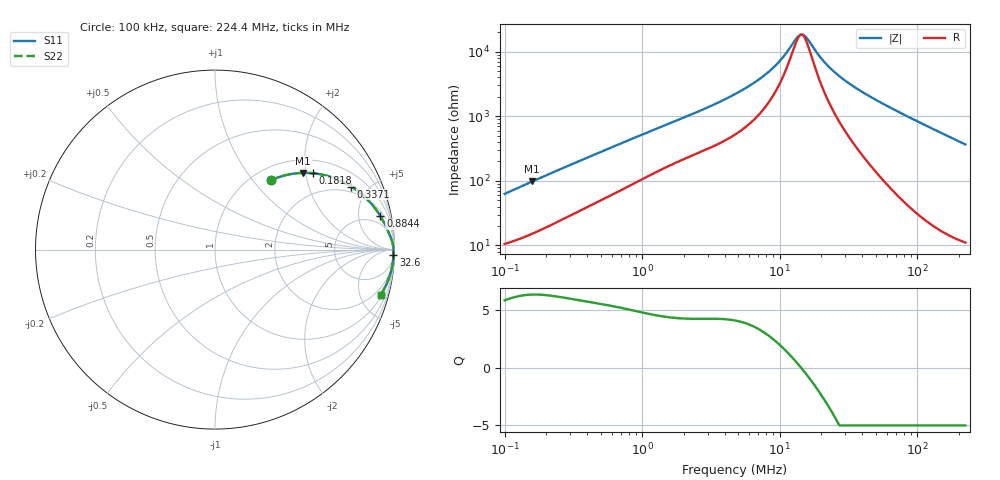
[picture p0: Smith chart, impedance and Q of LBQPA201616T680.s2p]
! LBQPA201616T680  S-PARAMETER MODEL  ( General Type )
! Model Generated by TAIYO YUDEN Corporation (http://www.ty-top.com)
! Version 1.0
! TAIYO YUDEN Control No. 191025NI43SB-FBB
! Copyright(c) 2019 TAIYO YUDEN CO.,LTD. All Rights Reserved.
! Product Description (link to TY-COMPAS)
! https://ds.yuden.co.jp/TYCOMPAS/or/detail?pn=LBQPA201616T680K&u=M
! Products Name : Inductors
! Characteristics :
!  Inductance : 68 uH , SRF(min) : 10 MHz , DC Resistance(max) : 9.1 Ohm
!  Rated Current : Saturation :130 mA , Temp Rise : 105 mA (20 degC)
!  Case Size : 2.0 x 1.6 / 0.079 x 0.063 [mm/inch] , Thickness : 1.6 / 0.063 [mm/inch]
!  (Conditions: Temperature = 25 degC , DC Bias Current/Voltage = 0A / 0V)
! External Node Assignments :
!  1  o---GGG---o  2
! GND o---------o GND
! Frequency Range : 0.1MHz  -  224.402193MHz  [ 402 STEP ]
# MHz S RI R 50
! Freq[MHz].  S11 Real  S11 Imag  S21 Real  S21 Imag  S12 Real  S12 Imag  S22 Real  S22 Imag
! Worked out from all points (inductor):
!   401 points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, 100 kHz to 224.4 MHz, reference 50 ohm
!   read as one part in series: L = 97.8 uH near 103.9 kHz
!   highest Q = 6.37 at 158.9 kHz (marker M1), where L = 96.9 uH
!   self-resonance near 14.22 MHz
!   S11 on the Smith chart (normalised r, x): 100 kHz: 1.21, +1.24; 181.8 kHz: 1.35, +2.20; 337.1 kHz: 1.66, +3.87; 884.4 kHz: 2.85, +9.15; 32.6 MHz: 10, -62; 224.4 MHz: 1.22, -7.31
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0.1  0.3117 0.3857  0.6883 -0.3857  0.6883 -0.3857  0.3117 0.3857
0.158877  0.4909 0.4275  0.5091 -0.4275  0.5091 -0.4275  0.4909 0.4275
0.181846  0.5459 0.4255  0.4541 -0.4255  0.4541 -0.4255  0.5459 0.4255
0.337122  0.7592 0.3512  0.2408 -0.3512  0.2408 -0.3512  0.7592 0.3512
0.364164  0.7795 0.3377  0.2205 -0.3377  0.2205 -0.3377  0.7795 0.3377
0.556677  0.8664 0.2607  0.1336 -0.2607  0.1336 -0.2607  0.8664 0.2607
0.884433  0.922 0.1857  0.078 -0.1857  0.078 -0.1857  0.922 0.1857
1.326154  0.9494 0.1349  0.0506 -0.1349  0.0506 -0.1349  0.9494 0.1349
2.868777  0.9778 0.0711  0.0222 -0.0711  0.0222 -0.0711  0.9778 0.0711
4.737111  0.9875 0.0431  0.0125 -0.0431  0.0125 -0.0431  0.9875 0.0431
6.575552  0.9912 0.0283  0.00884 -0.0283  0.00884 -0.0283  0.9912 0.0283
8.614263  0.993 0.0178  0.00703 -0.0178  0.00703 -0.0178  0.993 0.0178
10.44705  0.9938 0.0109  0.0062 -0.0109  0.0062 -0.0109  0.9938 0.0109
13.95267  0.9946 0.000991  0.00544 -0.000991  0.00544 -0.000991  0.9946 0.000991
14.50149  0.9946 -0.000312  0.00537 0.000312  0.00537 0.000312  0.9946 -0.000312
15.36545  0.9947 -0.00227  0.00529 0.00227  0.00529 0.00227  0.9947 -0.00227
17.25085  0.9948 -0.00623  0.00516 0.00623  0.00516 0.00623  0.9948 -0.00623
22.59938  0.9949 -0.0159  0.00509 0.0159  0.00509 0.0159  0.9949 -0.0159
32.60396  0.9945 -0.0312  0.00551 0.0312  0.00551 0.0312  0.9945 -0.0312
62.8214  0.9907 -0.0711  0.00926 0.0711  0.00926 0.0711  0.9907 -0.0711
121.0445  0.9748 -0.1411  0.0252 0.1411  0.0252 0.1411  0.9748 -0.1411
224.4022  0.924 -0.2503  0.076 0.2503  0.076 0.2503  0.924 -0.2503
